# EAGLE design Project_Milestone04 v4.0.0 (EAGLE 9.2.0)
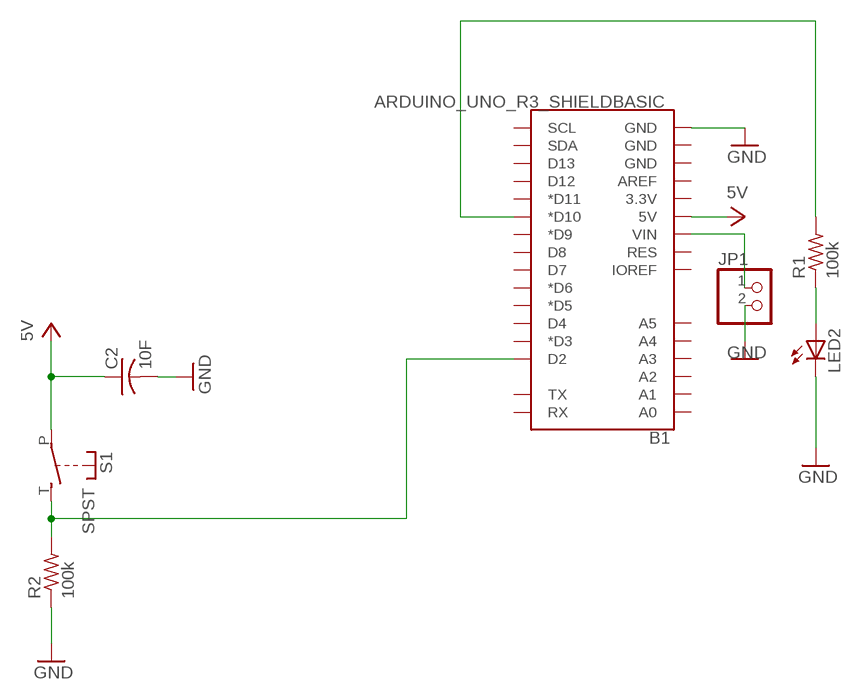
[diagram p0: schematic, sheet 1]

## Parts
B1  ARDUINO_UNO_R3_SHIELDBASIC  [UNO_R3_SHIELD]
C2  10F  C-USC0805  [C0805]
JP1  PINHD-1X2  [1X02]
LED2  LED5MM  [LED5MM]
R1  100k  R-US_0207/10  [0207/10]
R2  100k  R-US_0207/10  [0207/10]
S1  SPST  [JUDCOSPST]

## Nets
GND: B1.GND@0(GND) C2.2 JP1.2 LED2.K(C) R2.1
N$1: B1.VIN JP1.1
N$2: B1.D10(*D10) R1.2
N$4: LED2.A R1.1
N$7: B1.D2 R2.2 S1.T(S)
VCC: B1.5V C2.1 S1.P ; supply symbol labelled 5V
Unconnected: B1.3.3V B1.A0 B1.A1 B1.A2 B1.A3 B1.A4 B1.A5 B1.AREF B1.D3(*D3) B1.D4 B1.D5(*D5) B1.D6(*D6) B1.D7 B1.D8 B1.D9(*D9) B1.D11(*D11) B1.D12 B1.D13 B1.GND@1(GND) B1.GND@2(GND) B1.IOREF B1.RES B1.RX B1.SCL B1.SDA B1.TX

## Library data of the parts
B1 = SparkFun-Boards:ARDUINO_UNO_R3_SHIELD: Arduino R3 Shield Footprint Shield form compatible with the Arduino Uno R3. SparkFun Products: MG2639 Cellular Shield MIDI Shield R3 Stackable Headers Kit
C2 = adafruit:C-US: CAPACITOR, American symbol
JP1 = pinhead:PINHD-1X2: PIN HEADER
LED2 = adafruit:LED: LED
R1 R2 = rcl:R-US_: RESISTOR, American symbol; SPICEPREFIX: R
S1 = adafruit:SPST: Judco 50-0015-00

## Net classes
0 default: width 0.508 mm, drill 0.508 mm, clearance 0.508 mm

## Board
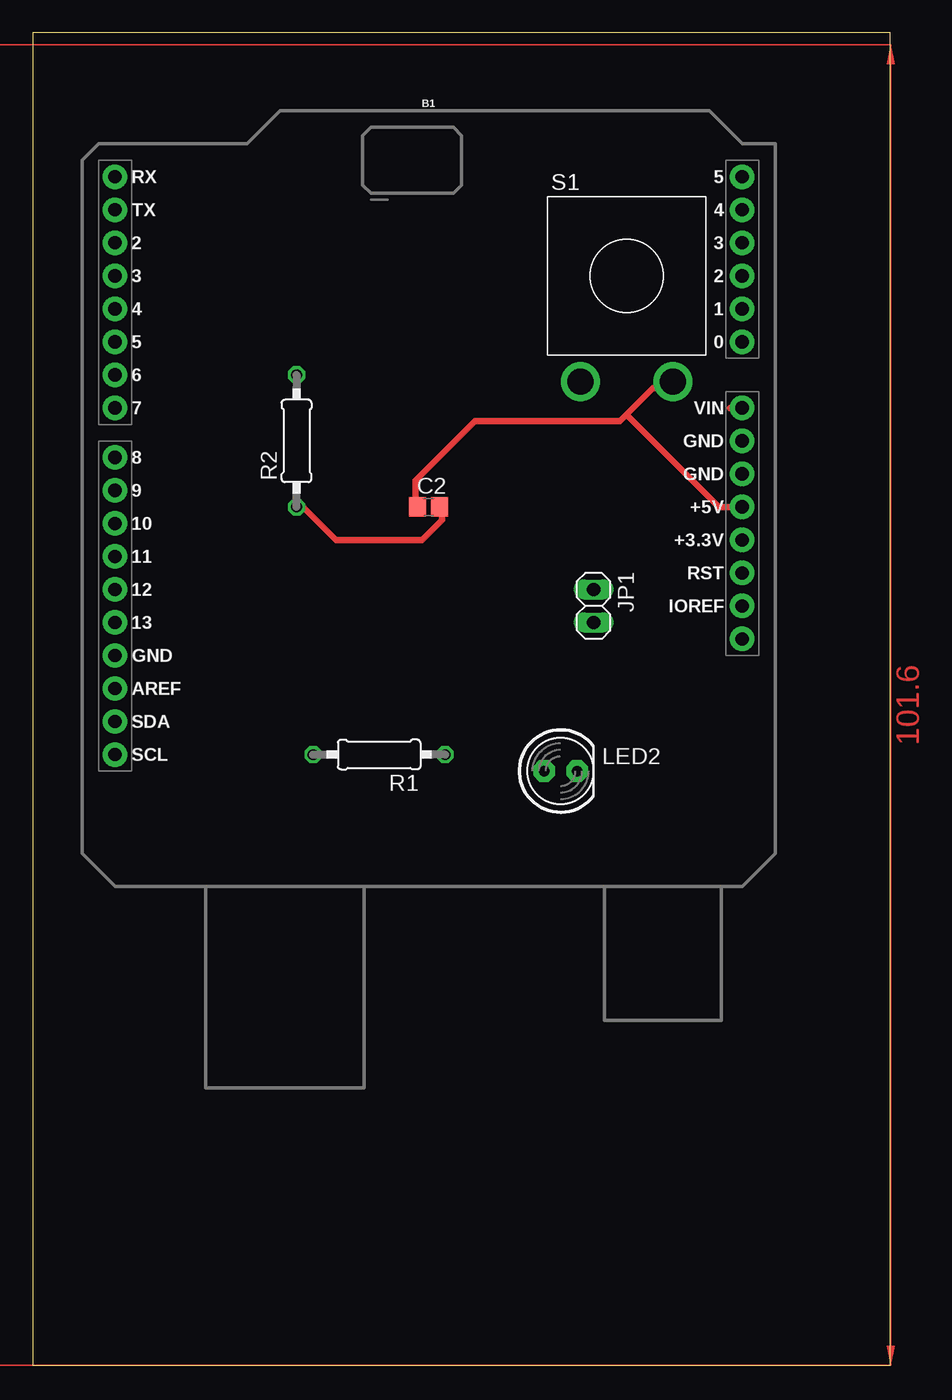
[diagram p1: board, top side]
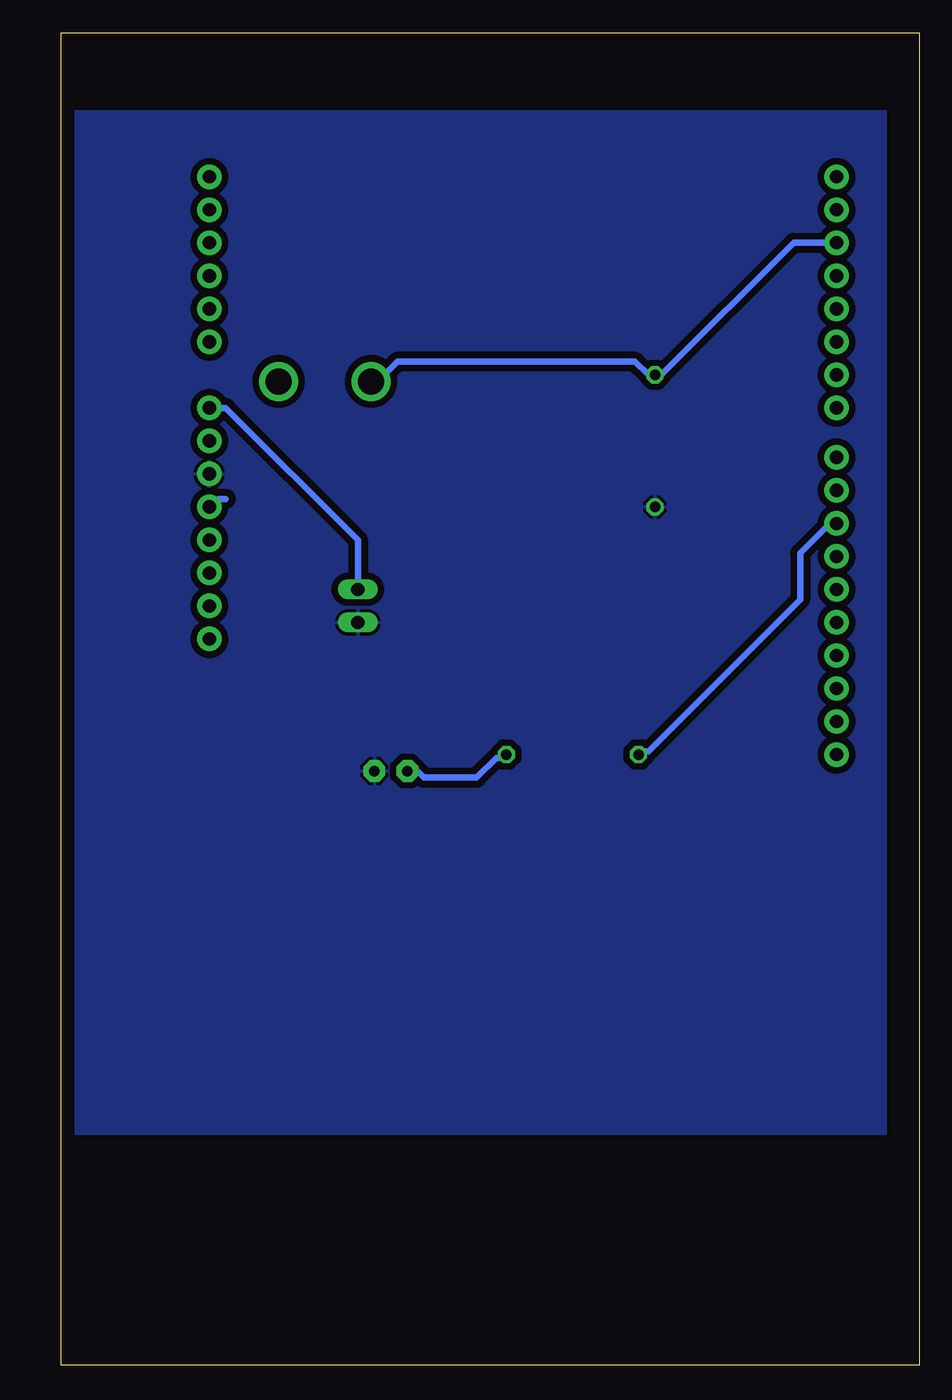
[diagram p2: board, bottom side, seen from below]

Size 66.02 x 102.54 mm. Coordinates in mm from the lower left corner, seen from the top.
Outline: 0,0 66.02,0 66.02,102.54 0,102.54 0,0
Copper layers (1*16): Top 0.035mm / dielectric 1.5mm / Bottom 0.035mm
Design rules "default": minimum track width 6mil, minimum drill 0.35mm, track to track 6mil, track to pad 6mil, pad to pad 6mil, via to via 6mil, smd to smd 6mil, copper to edge 40mil, drill to drill 6mil, minimum pad ring 10mil, minimum via ring 8mil, stop-mask expansion 4mil, vias tented up to drill 0mil, thermal gap 10mil

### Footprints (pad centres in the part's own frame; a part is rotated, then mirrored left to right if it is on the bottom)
UNO_R3_SHIELD = drill 1.016 pad 1.88: 3.3V 24.13,-2.54; 5V 24.13,0; A0 24.13,12.7; A1 24.13,15.24; A2 24.13,17.78; A3 24.13,20.32; A4 24.13,22.86; A5 24.13,25.4; AREF -24.13,-13.97; D2 -24.13,20.32; D3 -24.13,17.78; D4 -24.13,15.24; D5 -24.13,12.7; D6 -24.13,10.16; D7 -24.13,7.62; D8 -24.13,3.81; D9 -24.13,1.27; D10 -24.13,-1.27; D11 -24.13,-3.81; D12 -24.13,-6.35; D13 -24.13,-8.89; GND@0 24.13,2.54; GND@1 24.13,5.08; GND@2 -24.13,-11.43; IOREF 24.13,-7.62; NC 24.13,-10.16; RES 24.13,-5.08; RX -24.13,25.4; SCL -24.13,-19.05; SDA -24.13,-16.51; TX -24.13,22.86; VIN 24.13,7.62
C0805 = smd 1.3 x 1.5: 1 -0.85,0; 2 0.85,0
1X02 = drill 1.016 long: 1 -1.27,0; 2 1.27,0
LED5MM = drill 0.813 pad 1.676 octagon: A -1.27,0; K 1.27,0
0207/10 = drill 0.813 octagon: 1 -5.08,0; 2 5.08,0
JUDCOSPST = drill 2: P 3.556,-8.128; T -3.556,-8.128

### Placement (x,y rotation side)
B1  30.48,66.04 0 top
C2  30.48,66.04 0 top
JP1  43.18,58.42 270 top
LED2  40.64,45.72 0 top
R1  26.67,46.99 180 top
R2  20.32,71.12 90 top
S1  45.72,83.82 0 top

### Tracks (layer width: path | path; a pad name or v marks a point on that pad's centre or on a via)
GND
  Top 0.508: R2.1 20.83,66.04 23.37,63.5 29.97,63.5 31.5,65.02 31.5,66.04 C2.2
  pour Bottom: 2.54,96.52 2.54,17.78 66.04,17.78 66.04,96.52
N$1
  Top 0.508: B1.VIN 53.64,73.66 | 43.28,59.94 JP1.1
  Bottom 0.508: JP1.1 43.18,63.5 53.34,73.66 53.85,73.66 54.36,74.17 54.86,73.66 B1.VIN
N$2
  Top 0.508: 6.4,64.82 B1.D10
  Bottom 0.508: R1.2 21.34,47.24 20.83,47.24 9.14,58.93 9.14,62.48 6.6,65.02 B1.D10
N$4
  Bottom 0.508: 39.12,45.62 LED2.A 39.62,45.72 39.12,46.23 38.1,45.21 34.04,45.21 32.51,46.74 32,46.74 R1.1
N$7
  Bottom 0.508: 42.06,75.49 S1.T 41.66,75.69 40.13,77.22 21.84,77.22 20.83,76.2 R2.2 19.81,76.2 9.65,86.36 B1.D2
TOP
  pour Top: 66.04,17.78
VCC
  Top 0.508: 45.72,73.15 47.75,75.18 48.77,75.18 S1.P | 45.72,73.15 45.21,72.64 34.04,72.64 29.46,68.07 29.46,66.04 C2.1 | B1.5V 52.83,66.04 45.72,73.15
  Bottom 0.508: 53.34,66.65 53.95,66.65 54.56,66.04 B1.5V | 49.68,75.49 49.38,75.49 S1.P
(copper drawn outside any net)
  shapes: Top area x2

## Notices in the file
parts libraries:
SparkFun-Boards: Licensing: Creative Commons ShareAlike 4.0 International - https://creativecommons.org/licenses/by-sa/4.0
